(* Logix 5000 AddOnInstructionDefinition export YAI_Assy_155_117_EIP_Hz; software revision 21.03 *)

ADD_ON_INSTRUCTION YAI_Assy_155_117_EIP_Hz   (* revision 1.0, vendor Yaskawa America, Inc. *)
// YAI Assembly 155 and 117
// Help:
// This add-on instruction is for use with input assemblie 166 and output assemblies 116.
// Node_Input_Assy is defined as the node's input assembly integer array.
// Node_Output_Assy is defined as the node's output assembly integer array.
// Torque limit/reference, torque compensation and torque output variables are only available with A1000.
VAR_IN_OUT
   Node_Input_Assy : AB:ETHERNET_MODULE_INT_40Bytes:I:0; {required}   // Input assembly words
   Node_Output_Assy : AB:ETHERNET_MODULE_INT_8Bytes:O:0; {required}   // Output assembly words
END_VAR
VAR_INPUT
   RunFwd : BOOL; {visible}   // Forward run command
   RunRev : BOOL; {visible}   // Reverse run command
   MFI_3 : BOOL; {visible}   // Multi-function input 3
   MFI_4 : BOOL; {visible}   // Multi-function input 4
   MFI_5 : BOOL; {visible}   // Multi-function input 5
   MFI_6 : BOOL; {visible}   // Multi-function input 6
   MFI_7 : BOOL; {visible}   // Multi-function input 7
   MFI_8 : BOOL; {visible}   // Multi-function input 8
   External_Fault : BOOL;   // External fault command (EF0)
   FaultReset : BOOL; {visible}   // Fault reset command
   MFO_1 : BOOL; {visible}   // Multi-function output (M1-M2 for A/P1000, MA/MB/MC for V1000)
   MFO_2 : BOOL; {visible}   // Multi-function output (M3-M4 for A/P1000, P1 for V1000)
   MFO_3 : BOOL; {visible}   // Multi-function output (M5-M6 for A/P1000, P2 for V1000)
   Freq_Ref : REAL; {visible}   // Frequency reference command in Hz (xx.xx resolution)
   Digital_Output_Fault_Enable : BOOL;   // Bit to enable control of fault output relay over the network
END_VAR
VAR_OUTPUT
   Running : BOOL; {access Read Only, visible}   // Drive running forward status bit
   ZSP : BOOL; {access Read Only, visible}   // Drive zero speed status bit
   RunningRev : BOOL; {access Read Only, visible}   // Drive running reverse status bit
   Reset : BOOL; {access Read Only, visible}   // Drive reset command status bit
   At_Speed : BOOL; {access Read Only, visible}   // Drive at commanded speed status bit
   Ready : BOOL; {access Read Only, visible}   // Drive ready status bit
   Alarm : BOOL; {access Read Only, visible}   // Drive alarm status bit
   Faulted : BOOL; {access Read Only, visible}   // Drive faulted status bit
   OPE : BOOL; {access Read Only}   // OPE alarm/fault present
   UV : BOOL; {access Read Only}   // Drive in UV (undervoltage) state status bit
   NetCtrlStatus : BOOL; {access Read Only, visible}   // Drive network run source status bit (1 = source coming from network)
   MFO_1_Status : BOOL; {access Read Only, visible}   // Drive multi-function output 1 (M1-M2 for A/P1000, MA/MB/MC for V1000) status
   MFO_2_Status : BOOL; {access Read Only, visible}   // Drive multi-function output 1 (M3-M4 for A/P1000, P1 for V1000) status
   MFO_3_Status : BOOL; {access Read Only, visible}   // Drive multi-function output 1 (M5-M6 for A/P1000, P2 for V1000) status
   ZSV : BOOL; {access Read Only, visible}   // Drive zero servo completed status bit
   Motor_Speed : REAL; {access Read Only, visible}   // Motor speed in Hz (xx.xx resolution)
   Torque_Actual : REAL; {access Read Only, visible}   // Drive torque output in % (xxx.x resolution)
   PG1_Count : INT; {access Read Only}   // Encoder feedback count
   Freq_Cmd : REAL; {access Read Only, visible}   // Commanded frequency in Hz (xx.xx resolution)
   Output_Freq : REAL; {access Read Only, visible}   // Drive output frequency in Hz (xx.xx resolution)
   Output_Current : REAL; {access Read Only, visible}   // Drive output current in A (xxx.x resolution)
   Analog_Input_1_Level : REAL; {access Read Only}   // Analog input 1 level in % (xxx.x resolution)
   DC_Bus_Volt : INT; {access Read Only, visible}   // DC bus voltage in Vdc (xxx resolution)
   Analog_Input_3_Level : REAL; {access Read Only}   // Analog input 3 level in % (xxx.x resolution)
   Analog_Input_2_Level : REAL; {access Read Only}   // Analog input 2 level in % (xxx.x resolution)
   S1_Status : BOOL; {access Read Only}   // Digital input S1 status
   S2_Status : BOOL; {access Read Only}   // Digital input S2 status
   S3_Status : BOOL; {access Read Only}   // Digital input S3 status
   S4_Status : BOOL; {access Read Only}   // Digital input S4 status
   S5_Status : BOOL; {access Read Only}   // Digital input S5 status
   S6_Status : BOOL; {access Read Only}   // Digital input S6 status
   S7_Status : BOOL; {access Read Only}   // Digital input S7 status
   S8_Status : BOOL; {access Read Only}   // Digital input S8 status
   PG2_Count : INT;   // Encoder 2 feedback count
   UV_Alarm : BOOL; {access Read Only}   // Undervoltage alarm
   OV_Alarm : BOOL; {access Read Only}   // Overvoltage alarm
   OH_Alarm : BOOL; {access Read Only}   // Overheat alarm
   OH2_Alarm : BOOL; {access Read Only}   // Drive overheat alarm
   OL3_Alarm : BOOL; {access Read Only}   // Overtorque detection 1 alarm
   OL4_Alarm : BOOL; {access Read Only}   // Overtorque detection 2 alarm
   EF_Alarm : BOOL; {access Read Only}   // Run command error alarm
   bb_Alarm : BOOL; {access Read Only}   // Baseblock alarm
   EF3_Alarm : BOOL; {access Read Only}   // External fault 3 alarm
   EF4_Alarm : BOOL; {access Read Only}   // External fault 4 alarm
   EF5_Alarm : BOOL; {access Read Only}   // External fault 5 alarm
   EF6_Alarm : BOOL; {access Read Only}   // External fault 6 alarm
   EF7_Alarm : BOOL; {access Read Only}   // External fault 7 alarm
   EF8_Alarm : BOOL; {access Read Only}   // External fault 8 alarm
   FAN_Alarm : BOOL; {access Read Only}   // Cooling fan error alarm
   OS_Alarm : BOOL; {access Read Only}   // Overspeed alarm
   DEV_Alarm : BOOL; {access Read Only}   // Speed deviation alarm
   PGO_Alarm : BOOL; {access Read Only}   // Encoder feedback open alarm
   OPR_Alarm : BOOL; {access Read Only}   // Operator removed alarm
   CE_Alarm : BOOL; {access Read Only}   // Serial communication error alarm
   BUS_Alarm : BOOL; {access Read Only}   // BUS alarm
   CALL_Alarm : BOOL; {access Read Only}   // Serial communication timeout alarm
   OL1_Alarm : BOOL; {access Read Only}   // Motor overload alarm
   OL2_Alarm : BOOL; {access Read Only}   // Drive overload alarm
   EF0_Alarm : BOOL; {access Read Only}   // External fault 0 alarm
   RUN_Alarm : BOOL; {access Read Only}   // Motor 2 run command issued while running alarm
   UL3_Alarm : BOOL; {access Read Only}   // Undertorque detecxtion 1 alarm
   UL4_Alarm : BOOL; {access Read Only}   // Undertorque detection 2 alarm
   SE_Alarm : BOOL; {access Read Only}   // Modbus test failure alarm
   OH3_Alarm : BOOL; {access Read Only}   // Motor overload alarm
   FBL_Alarm : BOOL; {access Read Only}   // PID feedback loss alarm
   FBH_Alarm : BOOL; {access Read Only}   // PID feedback loss alarm
   DNE_Alarm : BOOL; {access Read Only}   // Drive not enabled alarm
END_VAR
VAR_INPUT
   Custom_Out_1 : INT;
   Custom_Out_2 : INT;
END_VAR
VAR
   FRef_Convert : DINT;
   FOut_Convert : REAL;
   FOut_Temp : REAL;
   TRef_Convert : INT;
   TComp_Convert : INT;
   TOut_Convert : REAL;
   TOut_Temp : REAL;
   IOut_Temp : REAL;
   IOut_Convert : REAL;
   AO1_Convert : INT;
   AO2_Convert : INT;
   Motor_Speed_Temp : REAL;
   Motor_Speed_Convert : REAL;
   Freq_Cmd_Temp : REAL;
   Freq_Cmd_Convert : REAL;
   AI1_Temp : REAL;
   AI1_Convert : REAL;
   AI2_Temp : REAL; {access None}
   AI2_Convert : REAL; {access None}
   AI3_Temp : REAL; {access None}
   AI3_Convert : REAL; {access None}
END_VAR

ROUTINE Logic   (* ladder *)
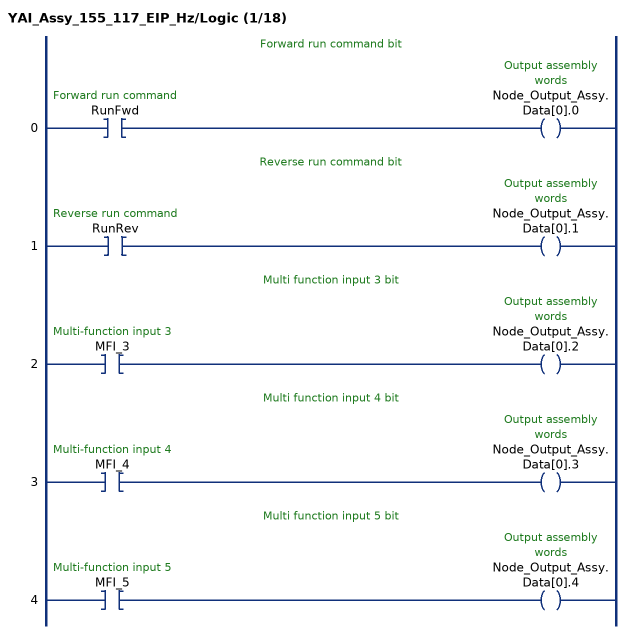
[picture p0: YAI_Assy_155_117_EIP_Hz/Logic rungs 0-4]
   // Forward run command bit
   0: XIC(RunFwd)OTE(Node_Output_Assy.Data[0].0);
   // Reverse run command bit
   1: XIC(RunRev)OTE(Node_Output_Assy.Data[0].1);
   // Multi function input 3 bit
   2: XIC(MFI_3)OTE(Node_Output_Assy.Data[0].2);
   // Multi function input 4 bit
   3: XIC(MFI_4)OTE(Node_Output_Assy.Data[0].3);
   // Multi function input 5 bit
   4: XIC(MFI_5)OTE(Node_Output_Assy.Data[0].4);
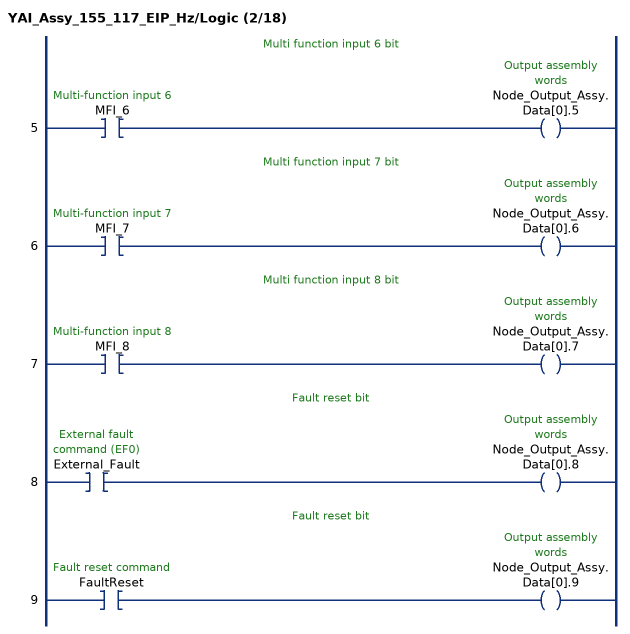
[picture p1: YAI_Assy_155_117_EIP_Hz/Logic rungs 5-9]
   // Multi function input 6 bit
   5: XIC(MFI_6)OTE(Node_Output_Assy.Data[0].5);
   // Multi function input 7 bit
   6: XIC(MFI_7)OTE(Node_Output_Assy.Data[0].6);
   // Multi function input 8 bit
   7: XIC(MFI_8)OTE(Node_Output_Assy.Data[0].7);
   // Fault reset bit
   8: XIC(External_Fault)OTE(Node_Output_Assy.Data[0].8);
   // Fault reset bit
   9: XIC(FaultReset)OTE(Node_Output_Assy.Data[0].9);
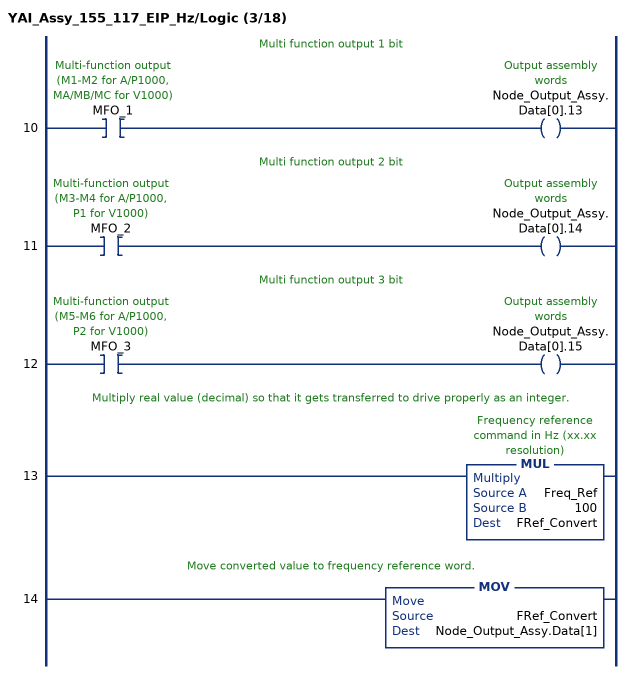
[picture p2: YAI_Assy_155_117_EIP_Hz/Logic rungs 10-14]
   // Multi function output 1 bit
   10: XIC(MFO_1)OTE(Node_Output_Assy.Data[0].13);
   // Multi function output 2 bit
   11: XIC(MFO_2)OTE(Node_Output_Assy.Data[0].14);
   // Multi function output 3 bit
   12: XIC(MFO_3)OTE(Node_Output_Assy.Data[0].15);
   // Multiply real value (decimal) so that it gets transferred to drive properly as an integer.
   13: MUL(Freq_Ref,100,FRef_Convert);
   // Move converted value to frequency reference word.
   14: MOV(FRef_Convert,Node_Output_Assy.Data[1]);
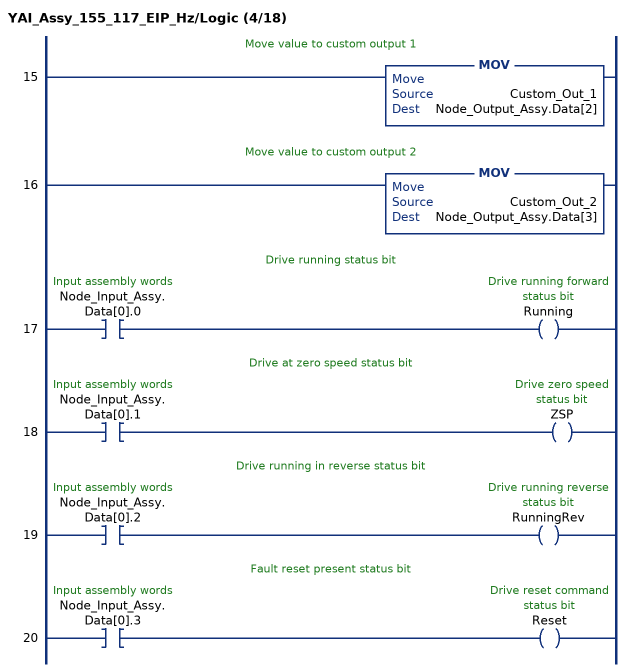
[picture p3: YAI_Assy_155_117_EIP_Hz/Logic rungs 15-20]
   // Move value to custom output 1
   15: MOV(Custom_Out_1,Node_Output_Assy.Data[2]);
   // Move value to custom output 2
   16: MOV(Custom_Out_2,Node_Output_Assy.Data[3]);
   // Drive running status bit
   17: XIC(Node_Input_Assy.Data[0].0)OTE(Running);
   // Drive at zero speed status bit
   18: XIC(Node_Input_Assy.Data[0].1)OTE(ZSP);
   // Drive running in reverse status bit
   19: XIC(Node_Input_Assy.Data[0].2)OTE(RunningRev);
   // Fault reset present status bit
   20: XIC(Node_Input_Assy.Data[0].3)OTE(Reset);
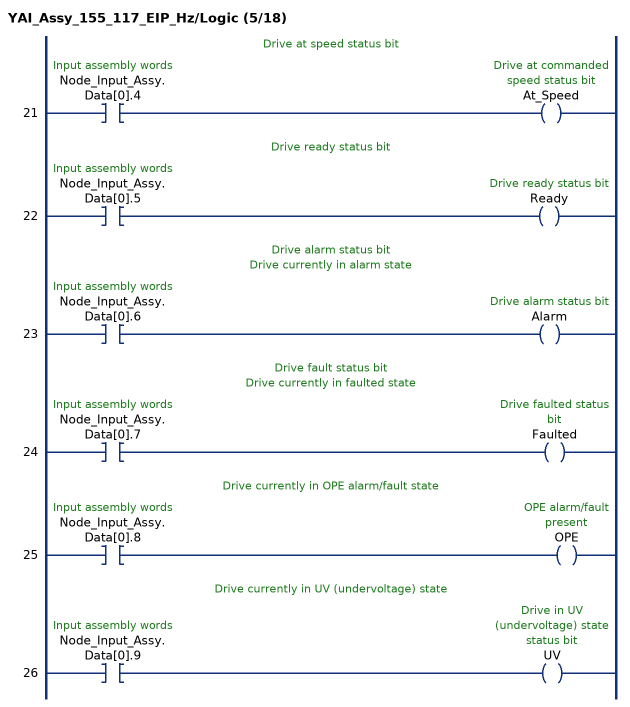
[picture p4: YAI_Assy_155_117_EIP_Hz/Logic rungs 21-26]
   // Drive at speed status bit
   21: XIC(Node_Input_Assy.Data[0].4)OTE(At_Speed);
   // Drive ready status bit
   22: XIC(Node_Input_Assy.Data[0].5)OTE(Ready);
   // Drive alarm status bit
   // Drive currently in alarm state
   23: XIC(Node_Input_Assy.Data[0].6)OTE(Alarm);
   // Drive fault status bit
   // Drive currently in faulted state
   24: XIC(Node_Input_Assy.Data[0].7)OTE(Faulted);
   // Drive currently in OPE alarm/fault state
   25: XIC(Node_Input_Assy.Data[0].8)OTE(OPE);
   // Drive currently in UV (undervoltage) state
   26: XIC(Node_Input_Assy.Data[0].9)OTE(UV);
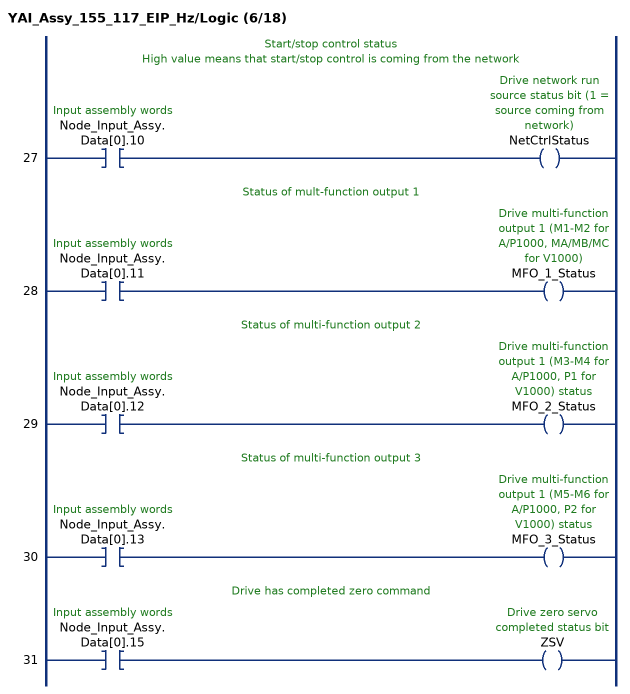
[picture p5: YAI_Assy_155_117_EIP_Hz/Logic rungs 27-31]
   // Start/stop control status
   // High value means that start/stop control is coming from the network
   27: XIC(Node_Input_Assy.Data[0].10)OTE(NetCtrlStatus);
   // Status of mult-function output 1
   28: XIC(Node_Input_Assy.Data[0].11)OTE(MFO_1_Status);
   // Status of multi-function output 2
   29: XIC(Node_Input_Assy.Data[0].12)OTE(MFO_2_Status);
   // Status of multi-function output 3
   30: XIC(Node_Input_Assy.Data[0].13)OTE(MFO_3_Status);
   // Drive has completed zero command
   31: XIC(Node_Input_Assy.Data[0].15)OTE(ZSV);
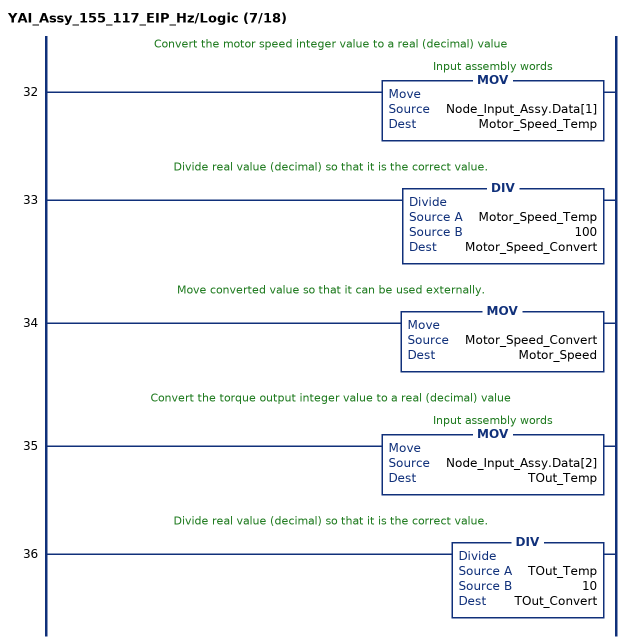
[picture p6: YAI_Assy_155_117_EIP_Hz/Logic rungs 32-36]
   // Convert the motor speed integer value to a real (decimal) value
   32: MOV(Node_Input_Assy.Data[1],Motor_Speed_Temp);
   // Divide real value (decimal) so that it is the correct value.
   33: DIV(Motor_Speed_Temp,100,Motor_Speed_Convert);
   // Move converted value so that it can be used externally.
   34: MOV(Motor_Speed_Convert,Motor_Speed);
   // Convert the torque output integer value to a real (decimal) value
   35: MOV(Node_Input_Assy.Data[2],TOut_Temp);
   // Divide real value (decimal) so that it is the correct value.
   36: DIV(TOut_Temp,10,TOut_Convert);
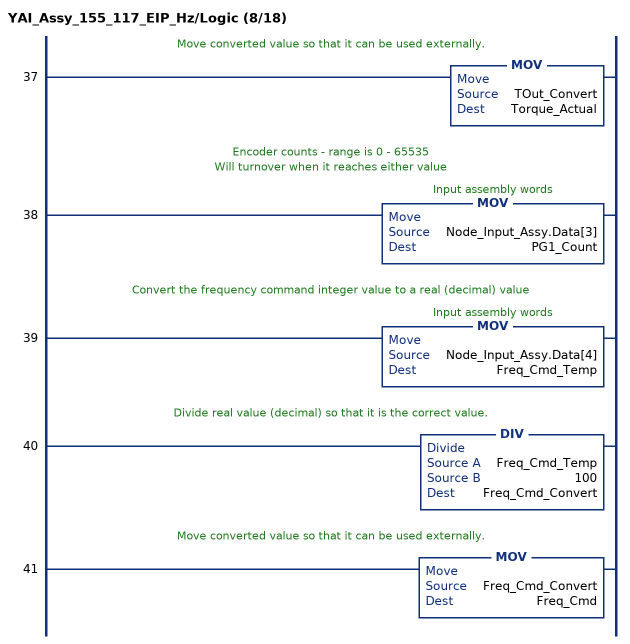
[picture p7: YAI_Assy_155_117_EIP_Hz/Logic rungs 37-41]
   // Move converted value so that it can be used externally.
   37: MOV(TOut_Convert,Torque_Actual);
   // Encoder counts - range is 0 - 65535
   // Will turnover when it reaches either value
   38: MOV(Node_Input_Assy.Data[3],PG1_Count);
   // Convert the frequency command integer value to a real (decimal) value
   39: MOV(Node_Input_Assy.Data[4],Freq_Cmd_Temp);
   // Divide real value (decimal) so that it is the correct value.
   40: DIV(Freq_Cmd_Temp,100,Freq_Cmd_Convert);
   // Move converted value so that it can be used externally.
   41: MOV(Freq_Cmd_Convert,Freq_Cmd);
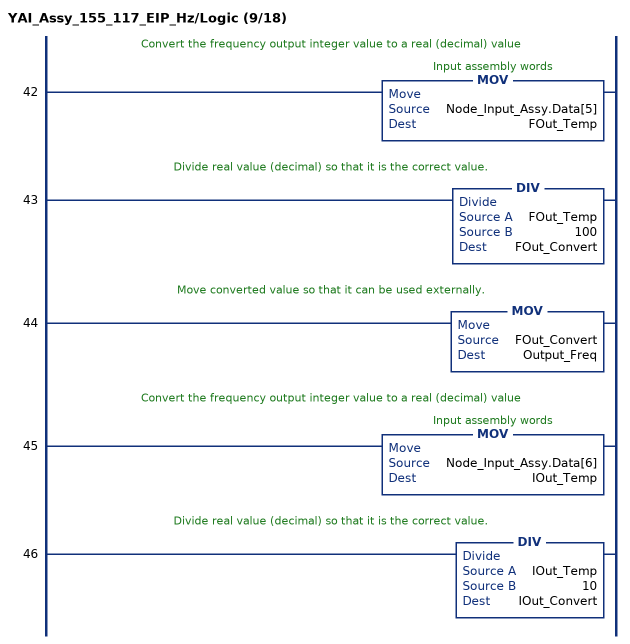
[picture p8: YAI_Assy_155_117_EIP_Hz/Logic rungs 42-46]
   // Convert the frequency output integer value to a real (decimal) value
   42: MOV(Node_Input_Assy.Data[5],FOut_Temp);
   // Divide real value (decimal) so that it is the correct value.
   43: DIV(FOut_Temp,100,FOut_Convert);
   // Move converted value so that it can be used externally.
   44: MOV(FOut_Convert,Output_Freq);
   // Convert the frequency output integer value to a real (decimal) value
   45: MOV(Node_Input_Assy.Data[6],IOut_Temp);
   // Divide real value (decimal) so that it is the correct value.
   46: DIV(IOut_Temp,10,IOut_Convert);
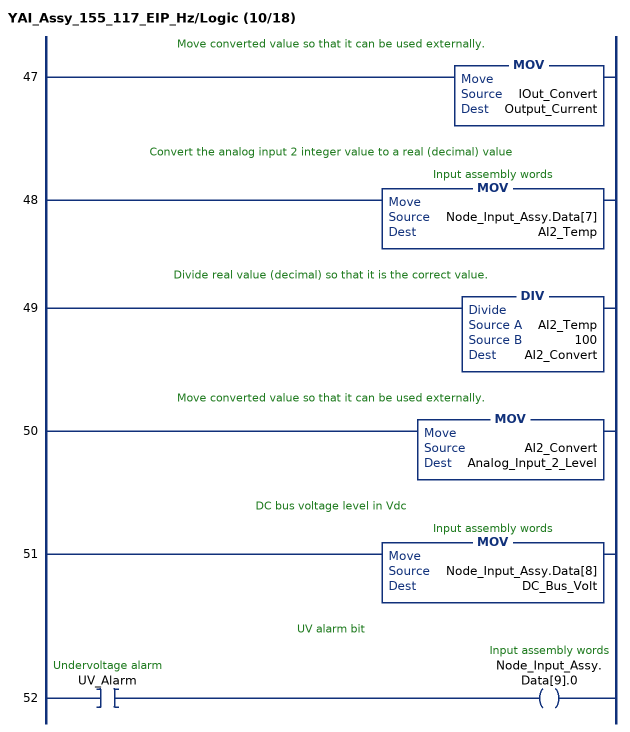
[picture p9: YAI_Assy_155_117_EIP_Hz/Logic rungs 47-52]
   // Move converted value so that it can be used externally.
   47: MOV(IOut_Convert,Output_Current);
   // Convert the analog input 2 integer value to a real (decimal) value
   48: MOV(Node_Input_Assy.Data[7],AI2_Temp);
   // Divide real value (decimal) so that it is the correct value.
   49: DIV(AI2_Temp,100,AI2_Convert);
   // Move converted value so that it can be used externally.
   50: MOV(AI2_Convert,Analog_Input_2_Level);
   // DC bus voltage level in Vdc
   51: MOV(Node_Input_Assy.Data[8],DC_Bus_Volt);
   // UV alarm bit
   52: XIC(UV_Alarm)OTE(Node_Input_Assy.Data[9].0);
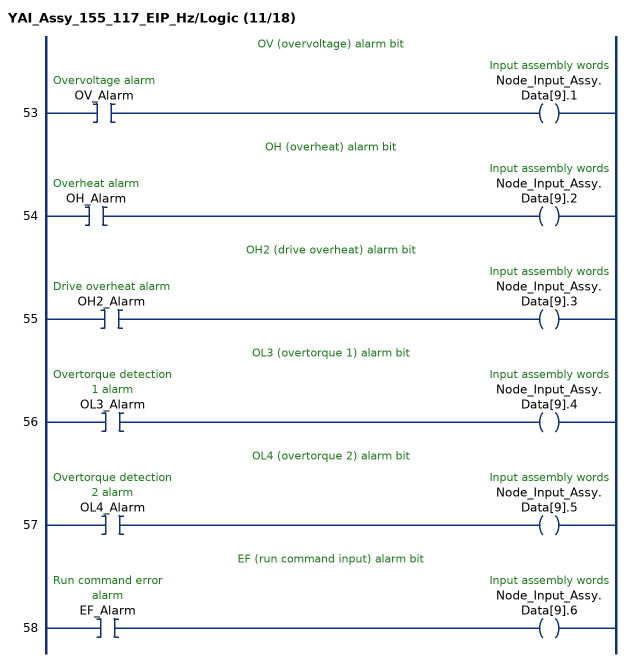
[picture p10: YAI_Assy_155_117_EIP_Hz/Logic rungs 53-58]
   // OV (overvoltage) alarm bit
   53: XIC(OV_Alarm)OTE(Node_Input_Assy.Data[9].1);
   // OH (overheat) alarm bit
   54: XIC(OH_Alarm)OTE(Node_Input_Assy.Data[9].2);
   // OH2 (drive overheat) alarm bit
   55: XIC(OH2_Alarm)OTE(Node_Input_Assy.Data[9].3);
   // OL3 (overtorque 1) alarm bit
   56: XIC(OL3_Alarm)OTE(Node_Input_Assy.Data[9].4);
   // OL4 (overtorque 2) alarm bit
   57: XIC(OL4_Alarm)OTE(Node_Input_Assy.Data[9].5);
   // EF (run command input) alarm bit
   58: XIC(EF_Alarm)OTE(Node_Input_Assy.Data[9].6);
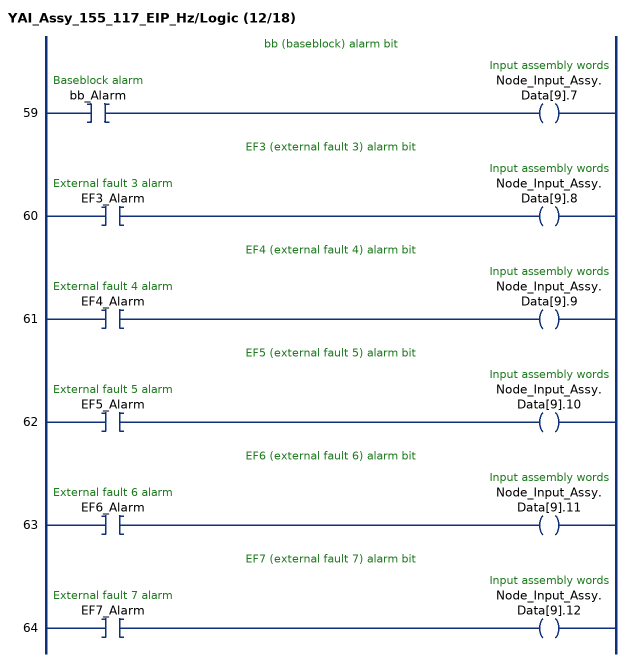
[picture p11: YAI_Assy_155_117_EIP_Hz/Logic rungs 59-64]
   // bb (baseblock) alarm bit
   59: XIC(bb_Alarm)OTE(Node_Input_Assy.Data[9].7);
   // EF3 (external fault 3) alarm bit
   60: XIC(EF3_Alarm)OTE(Node_Input_Assy.Data[9].8);
   // EF4 (external fault 4) alarm bit
   61: XIC(EF4_Alarm)OTE(Node_Input_Assy.Data[9].9);
   // EF5 (external fault 5) alarm bit
   62: XIC(EF5_Alarm)OTE(Node_Input_Assy.Data[9].10);
   // EF6 (external fault 6) alarm bit
   63: XIC(EF6_Alarm)OTE(Node_Input_Assy.Data[9].11);
   // EF7 (external fault 7) alarm bit
   64: XIC(EF7_Alarm)OTE(Node_Input_Assy.Data[9].12);
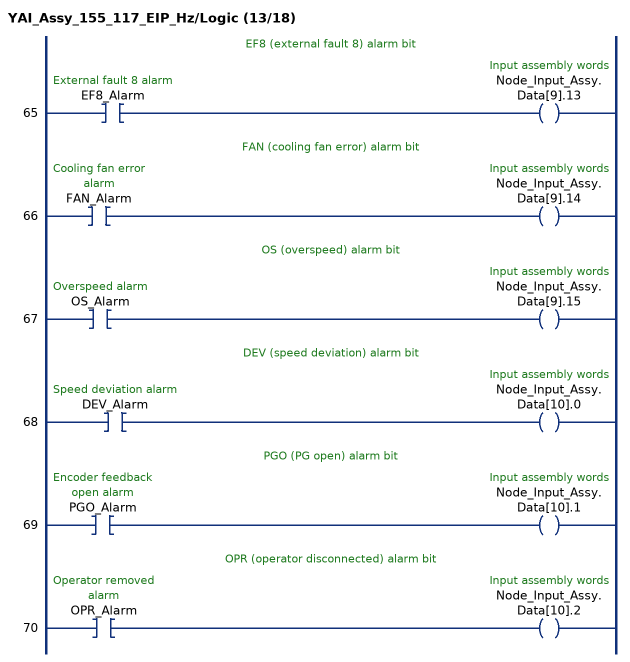
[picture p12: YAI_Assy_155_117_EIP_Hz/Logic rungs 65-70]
   // EF8 (external fault 8) alarm bit
   65: XIC(EF8_Alarm)OTE(Node_Input_Assy.Data[9].13);
   // FAN (cooling fan error) alarm bit
   66: XIC(FAN_Alarm)OTE(Node_Input_Assy.Data[9].14);
   // OS (overspeed) alarm bit
   67: XIC(OS_Alarm)OTE(Node_Input_Assy.Data[9].15);
   // DEV (speed deviation) alarm bit
   68: XIC(DEV_Alarm)OTE(Node_Input_Assy.Data[10].0);
   // PGO (PG open) alarm bit
   69: XIC(PGO_Alarm)OTE(Node_Input_Assy.Data[10].1);
   // OPR (operator disconnected) alarm bit
   70: XIC(OPR_Alarm)OTE(Node_Input_Assy.Data[10].2);
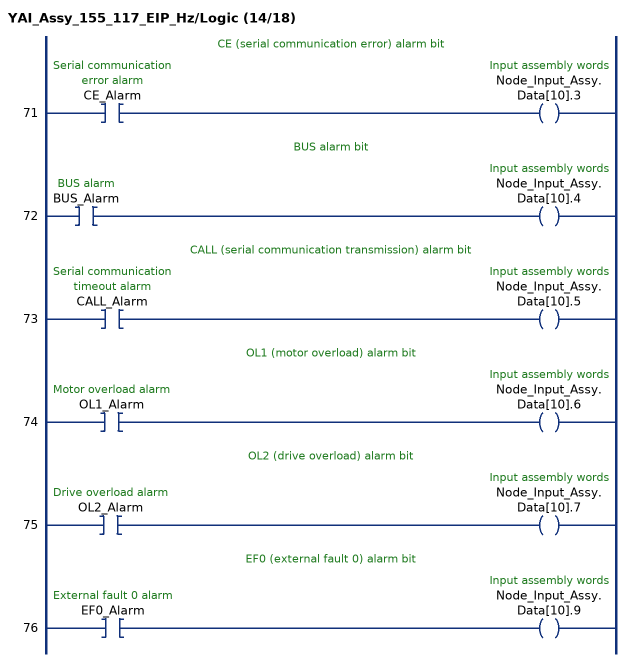
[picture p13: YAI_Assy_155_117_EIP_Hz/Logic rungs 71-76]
   // CE (serial communication error) alarm bit
   71: XIC(CE_Alarm)OTE(Node_Input_Assy.Data[10].3);
   // BUS alarm bit
   72: XIC(BUS_Alarm)OTE(Node_Input_Assy.Data[10].4);
   // CALL (serial communication transmission) alarm bit
   73: XIC(CALL_Alarm)OTE(Node_Input_Assy.Data[10].5);
   // OL1 (motor overload) alarm bit
   74: XIC(OL1_Alarm)OTE(Node_Input_Assy.Data[10].6);
   // OL2 (drive overload) alarm bit
   75: XIC(OL2_Alarm)OTE(Node_Input_Assy.Data[10].7);
   // EF0 (external fault 0) alarm bit
   76: XIC(EF0_Alarm)OTE(Node_Input_Assy.Data[10].9);
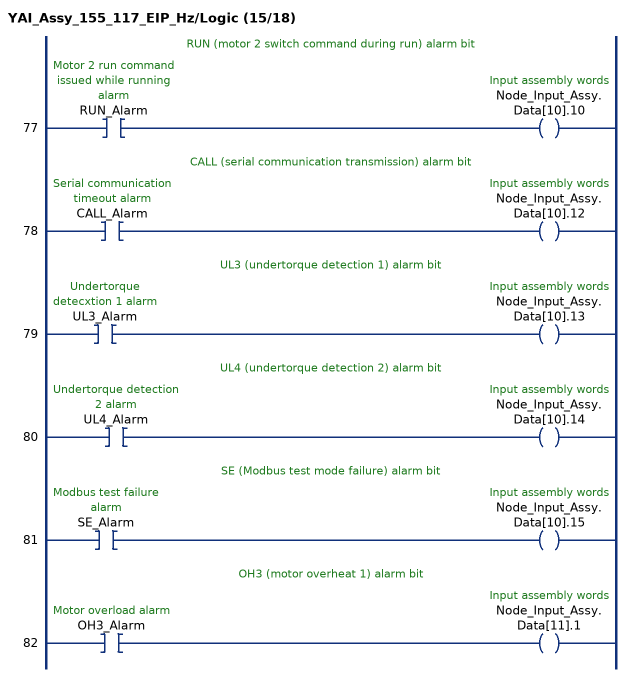
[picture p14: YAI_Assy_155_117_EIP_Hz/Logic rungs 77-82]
   // RUN (motor 2 switch command during run) alarm bit
   77: XIC(RUN_Alarm)OTE(Node_Input_Assy.Data[10].10);
   // CALL (serial communication transmission) alarm bit
   78: XIC(CALL_Alarm)OTE(Node_Input_Assy.Data[10].12);
   // UL3 (undertorque detection 1) alarm bit
   79: XIC(UL3_Alarm)OTE(Node_Input_Assy.Data[10].13);
   // UL4 (undertorque detection 2) alarm bit
   80: XIC(UL4_Alarm)OTE(Node_Input_Assy.Data[10].14);
   // SE (Modbus test mode failure) alarm bit
   81: XIC(SE_Alarm)OTE(Node_Input_Assy.Data[10].15);
   // OH3 (motor overheat 1) alarm bit
   82: XIC(OH3_Alarm)OTE(Node_Input_Assy.Data[11].1);
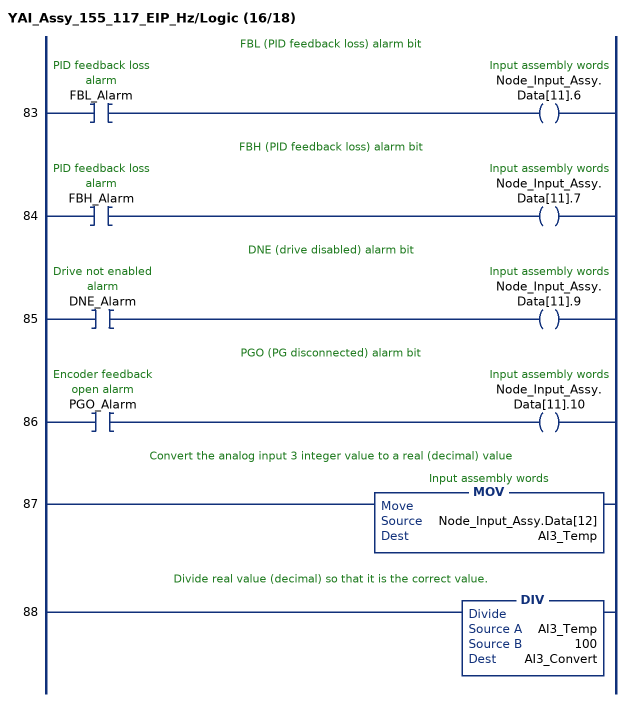
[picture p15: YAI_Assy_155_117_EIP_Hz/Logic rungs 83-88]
   // FBL (PID feedback loss) alarm bit
   83: XIC(FBL_Alarm)OTE(Node_Input_Assy.Data[11].6);
   // FBH (PID feedback loss) alarm bit
   84: XIC(FBH_Alarm)OTE(Node_Input_Assy.Data[11].7);
   // DNE (drive disabled) alarm bit
   85: XIC(DNE_Alarm)OTE(Node_Input_Assy.Data[11].9);
   // PGO (PG disconnected) alarm bit
   86: XIC(PGO_Alarm)OTE(Node_Input_Assy.Data[11].10);
   // Convert the analog input 3 integer value to a real (decimal) value
   87: MOV(Node_Input_Assy.Data[12],AI3_Temp);
   // Divide real value (decimal) so that it is the correct value.
   88: DIV(AI3_Temp,100,AI3_Convert);
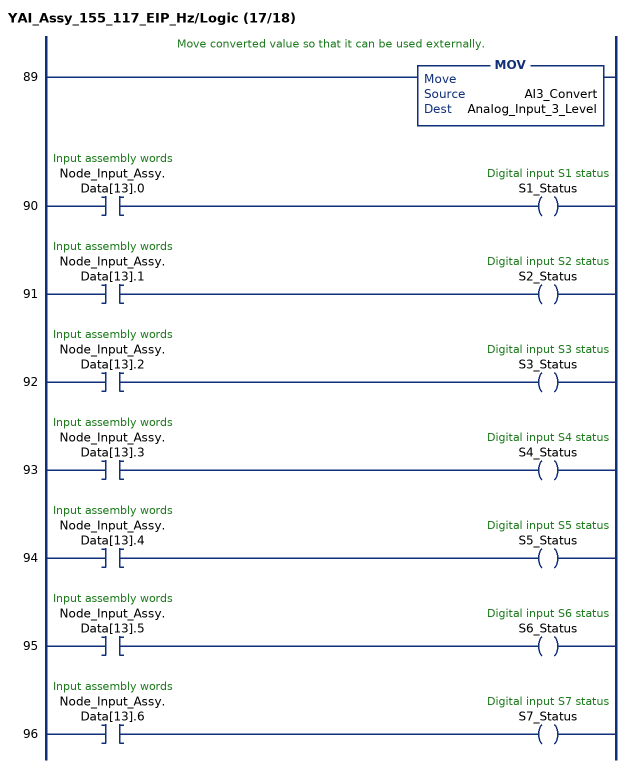
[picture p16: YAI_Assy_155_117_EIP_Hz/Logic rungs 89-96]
   // Move converted value so that it can be used externally.
   89: MOV(AI3_Convert,Analog_Input_3_Level);
   90: XIC(Node_Input_Assy.Data[13].0)OTE(S1_Status);
   91: XIC(Node_Input_Assy.Data[13].1)OTE(S2_Status);
   92: XIC(Node_Input_Assy.Data[13].2)OTE(S3_Status);
   93: XIC(Node_Input_Assy.Data[13].3)OTE(S4_Status);
   94: XIC(Node_Input_Assy.Data[13].4)OTE(S5_Status);
   95: XIC(Node_Input_Assy.Data[13].5)OTE(S6_Status);
   96: XIC(Node_Input_Assy.Data[13].6)OTE(S7_Status);
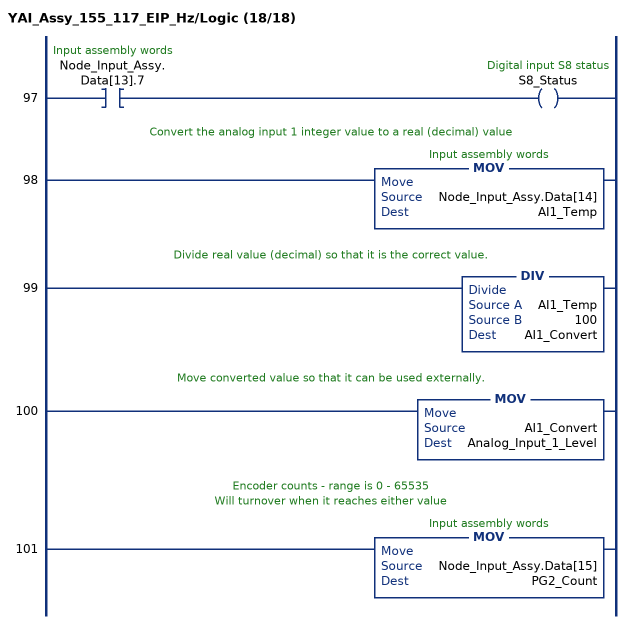
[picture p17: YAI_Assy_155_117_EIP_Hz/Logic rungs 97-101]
   97: XIC(Node_Input_Assy.Data[13].7)OTE(S8_Status);
   // Convert the analog input 1 integer value to a real (decimal) value
   98: MOV(Node_Input_Assy.Data[14],AI1_Temp);
   // Divide real value (decimal) so that it is the correct value.
   99: DIV(AI1_Temp,100,AI1_Convert);
   // Move converted value so that it can be used externally.
   100: MOV(AI1_Convert,Analog_Input_1_Level);
   // Encoder counts - range is 0 - 65535
   // Will turnover when it reaches either value
   101: MOV(Node_Input_Assy.Data[15],PG2_Count);
END_ROUTINE
END_ADD_ON_INSTRUCTION
